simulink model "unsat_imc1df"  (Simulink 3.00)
settings: Solver=ode45  SolverMode=SingleTasking  StartTime=0.0  StopTime=50  MaxStep=st_size  RelTol=1e-5  AbsTol=1e-6
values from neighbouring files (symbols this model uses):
  Disturb = Setpoint    [mimo_MSF1DF_sim.m]    (also in mimo_MSF2DF_sim.m)
  Setpoint = zeros(1,n)    [mimo_MSF1DF_sim.m]    (also in mimo_MSF2DF_sim.m)
undefined symbols (not defined in the file or in its folder): denCs, denMs, denPd, denPs, Mdelay, numCs, numMs, numPd, numPs, Pdelay

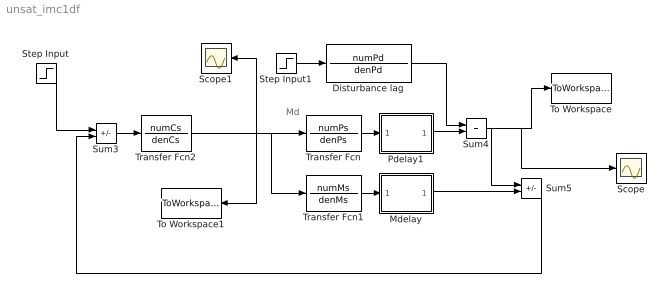
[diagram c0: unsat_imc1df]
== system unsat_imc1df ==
  note: Md
  Disturbance lag : TransferFcn  Numerator=numPd  Denominator=denPd
  Mdelay : Subsystem
  Pdelay1 : Subsystem
  Scope : Scope
  Scope1 : Scope
  Step Input : Step  Time=0  Before=0  After=Setpoint  SampleTime=0
  Step Input1 : Step  Time=0  Before=0  After=Disturb  SampleTime=0
  Sum3 : Sum  Inputs=+-  SaturateOnIntegerOverflow=on
  Sum4 : Sum  Inputs=++  SaturateOnIntegerOverflow=on
  Sum5 : Sum  Inputs=+-  SaturateOnIntegerOverflow=on
  To Workspace : ToWorkspace  VariableName=simout  SampleTime=-1  SaveFormat=Matrix
  To Workspace1 : ToWorkspace  VariableName=effort  SampleTime=-1  SaveFormat=Matrix
  Transfer Fcn : TransferFcn  Numerator=numPs  Denominator=denPs
  Transfer Fcn1 : TransferFcn  Numerator=numMs  Denominator=denMs
  Transfer Fcn2 : TransferFcn  Numerator=numCs  Denominator=denCs
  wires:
  Sum3/1 -> Transfer Fcn2/1
  Disturbance lag/1 -> Sum4/1
  Pdelay1/1(Out1) -> Sum4/2
  Transfer Fcn/1 -> Pdelay1/1(In1)
  Step Input1/1 -> Disturbance lag/1
  Step Input/1 -> Sum3/1
  Transfer Fcn1/1 -> Mdelay/1(In1)
  Sum4/1 -> Sum5/1, To Workspace/1, Scope/1
  Mdelay/1(Out1) -> Sum5/2
  Sum5/1 -> Sum3/2
  Transfer Fcn2/1 -> Transfer Fcn/1, Transfer Fcn1/1, Scope1/1, To Workspace1/1

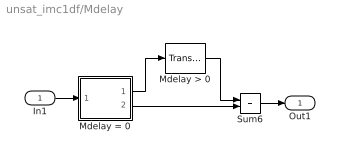
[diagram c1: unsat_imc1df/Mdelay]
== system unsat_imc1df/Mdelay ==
  In1 : Inport  Port=1  PortWidth=-1  SampleTime=-1  DataType=auto
  Mdelay > 0 : TransportDelay  DelayTime=Mdelay  InitialInput=0  BufferSize=1024
  Mdelay = 0 : Subsystem  Description=pass input signal through out1 if condition is true.
  Sum6 : Sum  Inputs=++  SaturateOnIntegerOverflow=on
  Out1 : Outport  Port=1
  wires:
  Mdelay = 0/1(Out2) -> Mdelay > 0/1
  Mdelay > 0/1 -> Sum6/1
  Mdelay = 0/2(Out1) -> Sum6/2
  In1/1 -> Mdelay = 0/1(In)
  Sum6/1 -> Out1/1

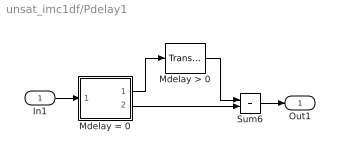
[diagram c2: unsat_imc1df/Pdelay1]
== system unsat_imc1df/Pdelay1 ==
  In1 : Inport  Port=1  PortWidth=-1  SampleTime=-1  DataType=auto
  Mdelay > 0 : TransportDelay  DelayTime=Pdelay  InitialInput=0  BufferSize=1024
  Mdelay = 0 : Subsystem  Description=pass input signal through out1 if condition is true.
  Sum6 : Sum  Inputs=++  SaturateOnIntegerOverflow=on
  Out1 : Outport  Port=1
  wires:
  Mdelay = 0/1(Out2) -> Mdelay > 0/1
  Mdelay > 0/1 -> Sum6/1
  Mdelay = 0/2(Out1) -> Sum6/2
  In1/1 -> Mdelay = 0/1(In)
  Sum6/1 -> Out1/1

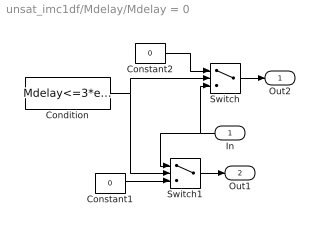
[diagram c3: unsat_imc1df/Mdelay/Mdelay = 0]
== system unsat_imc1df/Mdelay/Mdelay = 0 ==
  In : Inport  Orientation=left  Port=1  PortWidth=-1  SampleTime=-1  DataType=auto
  Condition : Constant  Value=Mdelay<=3*eps
  Constant1 : Constant  Value=0
  Constant2 : Constant  Value=0
  Switch : Switch  Threshold=1
  Switch1 : Switch  Threshold=1
  Out2 : Outport  Port=1  InitialOutput=0
  Out1 : Outport  Port=2  InitialOutput=0
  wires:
  In/1 -> Switch/3, Switch1/1
  Condition/1 -> Switch1/2, Switch/2
  Constant1/1 -> Switch1/3
  Constant2/1 -> Switch/1
  Switch/1 -> Out2/1
  Switch1/1 -> Out1/1

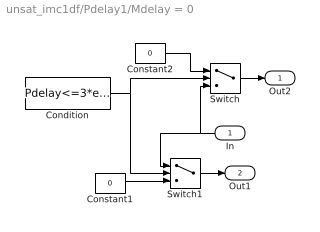
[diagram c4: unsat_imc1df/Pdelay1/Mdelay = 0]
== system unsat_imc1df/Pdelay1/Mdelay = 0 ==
  In : Inport  Orientation=left  Port=1  PortWidth=-1  SampleTime=-1  DataType=auto
  Condition : Constant  Value=Pdelay<=3*eps
  Constant1 : Constant  Value=0
  Constant2 : Constant  Value=0
  Switch : Switch  Threshold=1
  Switch1 : Switch  Threshold=1
  Out2 : Outport  Port=1  InitialOutput=0
  Out1 : Outport  Port=2  InitialOutput=0
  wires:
  In/1 -> Switch/3, Switch1/1
  Condition/1 -> Switch1/2, Switch/2
  Constant1/1 -> Switch1/3
  Constant2/1 -> Switch/1
  Switch/1 -> Out2/1
  Switch1/1 -> Out1/1
